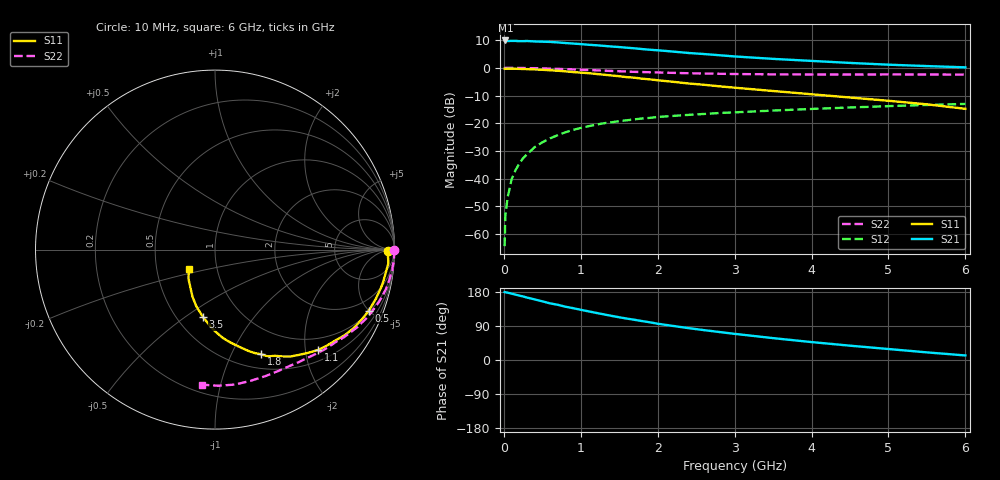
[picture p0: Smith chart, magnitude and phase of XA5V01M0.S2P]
! SIEMENS Discrete & RF Semiconductors
! BFY180
! Si NPN RF Bipolar Junction Transistor in MICRO-X
! VCE = 5 V  IC = 1 mA
! Common Emitter S-Parameters:  May  1997
# GHz  S  MA  R  50
!  f  S11  S21  S12  S22
! GHz  MAG  ANG  MAG  ANG  MAG  ANG  MAG  ANG
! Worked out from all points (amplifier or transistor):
!   36 points, 10 MHz to 6 GHz, reference 50 ohm
!   highest |S21| = 9.9 dB at 20 MHz (marker M1)
!   |S21| within 3 dB of that: start of sweep to 1.757 GHz
!   unconditionally stable (mu >= 1): 4.061 GHz to end of sweep
!   at 250 MHz: K = 0.06, MSG = 21.1 dB, |S12| = -32.7 dB
!   at 1.4 GHz: K = 0.49, MSG = 13.7 dB, |S12| = -19.7 dB
!   at 6 GHz: K = 1.05, MAG = 5.3 dB, |S12| = -13.0 dB
!   S11 on the Smith chart (normalised r, x): 10 MHz: 55, -11; 500 MHz: 1.10, -5.01; 1.1 GHz: 0.72, -2.27; 1.8 GHz: 0.67, -1.31; 3.5 GHz: 0.67, -0.59; 6 GHz: 0.73, -0.16
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0.01  0.9654 -0.4  3.066 179.3  0.0006 84.0  0.9952 -0.2
0.02  0.9597 -1.0  3.127 178.7  0.0022 86.4  0.9999 -0.5
0.05  0.964 -2.0  3.051 177.6  0.0046 86.3  0.9985 -1.3
0.1  0.9693 -4.5  3.068 175.2  0.0096 88.2  0.9982 -2.6
0.15  0.9628 -6.6  3.071 172.6  0.014 85.2  0.9974 -4.0
0.25  0.9536 -11.1  3.036 167.7  0.0233 83.3  0.9945 -6.6
0.3  0.9487 -13.1  3.058 164.8  0.0273 80.7  0.9896 -8.0
0.5  0.9226 -21.6  2.971 154.8  0.0451 74.6  0.9777 -13.0
0.6  0.9049 -25.6  2.944 149.5  0.0531 72.2  0.968 -15.4
0.8  0.8647 -33.6  2.81 140.6  0.0685 66.4  0.9468 -20.1
1.1  0.8016 -44.2  2.614 128.4  0.0881 59.1  0.9133 -26.5
1.2  0.7764 -47.7  2.563 124.3  0.0943 56.7  0.9033 -28.6
1.5  0.7057 -57.6  2.378 112.7  0.1091 50.8  0.8684 -34.2
1.8  0.6373 -66.2  2.183 102.6  0.1219 46.2  0.8401 -39.0
2.2  0.5598 -75.8  1.968 89.9  0.1355 40.4  0.8121 -45.2
2.4  0.5222 -80.9  1.858 84.1  0.1414 38.1  0.7992 -48.0
2.8  0.4643 -88.7  1.691 73.9  0.1528 34.2  0.7822 -53.2
3.5  0.3819 -100.1  1.454 57.7  0.1693 28.2  0.7632 -62.0
4  0.3334 -108.1  1.335 47.3  0.181 24.1  0.7586 -68.4
4.5  0.2912 -115.5  1.228 37.8  0.1924 20.2  0.7575 -75.0
5.5  0.2193 -132.4  1.077 20.1  0.2134 12.5  0.7589 -88.6
6  0.1818 -143.4  1.022 12.0  0.2233 8.2  0.7559 -95.5
